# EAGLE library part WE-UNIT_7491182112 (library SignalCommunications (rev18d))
WE-UNIT Off-Line Transformer Characteristics Nominal input voltage: 125–375 VDC (85–265 VAC) Output power 3 W and 9 W Operating temperature: –40 °C to +125 °C Clearance and creepage distance 6 mm min. Insulation test voltage: 4 kVAC, 1 Minute Design compliant to EN 61558-2-16: reinforced insulation; except 749 118 10 xx: Basic insulation Applications Designed for Tiny Switch ICs from Power Integration and NCP101x or 105x of ON Semiconductor For SMPS with universal input from 85 VAC up to 265 VAC Details see: http://katalog.we-online.de/en/pbs/WE-UNIT?m Updated by Dan Xu 2014-07-11 2014 (C) Wurth Elektronik
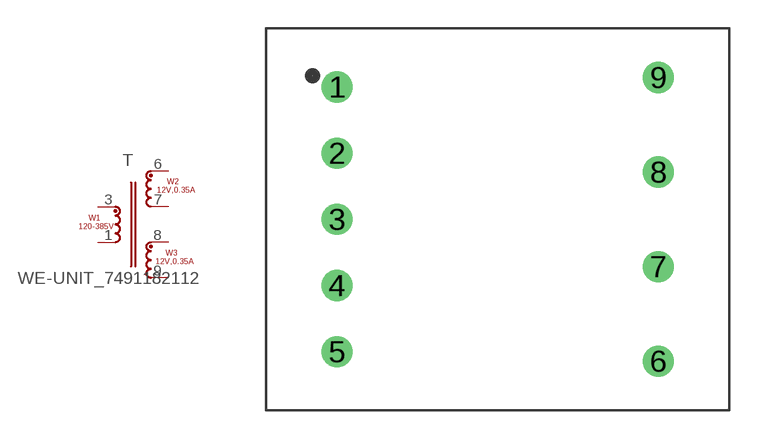
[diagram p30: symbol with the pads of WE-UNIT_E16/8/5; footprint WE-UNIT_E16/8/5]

Designator prefix T

## WE-UNIT_7491182112_7491182112, WE-UNIT_7491182112_7491182124, WE-UNIT_7491182112_749118215  [WE-UNIT_E16/8/5]
1  6  pas
3  1  pas
6  2  pas
7  3  pas
8  4  pas
9  5  pas

## Footprint WE-UNIT_E16/8/5 (pad centres in mm)
Transformer, E16/8/5 THT Horizontal 9 Pin
drill 1.1: 1 -8.5,7; 2 -8.5,3.5; 3 -8.5,0; 4 -8.5,-3.5; 5 -8.5,-7; 6 8.5,-7.5; 7 8.5,-2.5; 8 8.5,2.5; 9 8.5,7.5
